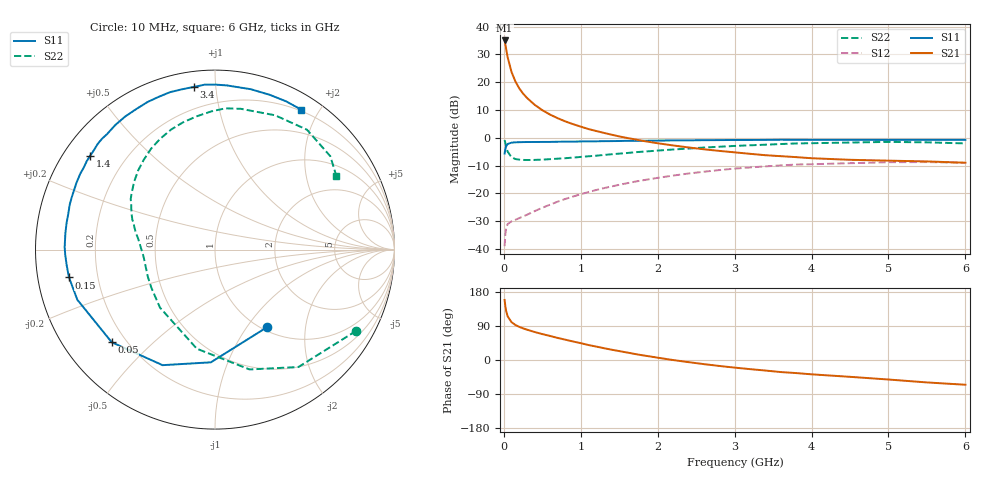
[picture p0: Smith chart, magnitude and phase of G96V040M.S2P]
! SIEMENS Small Signal Semiconductors
! BFG235
! Si NPN RF Bipolar Junction Transistor in SOT223
! VCE = 6 V  IC = 40 mA
! Common Emitter S-Parameters:  July  1994
# GHz  S  MA  R  50
!  f  S11  S21  S12  S22
! GHz  MAG  ANG  MAG  ANG  MAG  ANG  MAG  ANG
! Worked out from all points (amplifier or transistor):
!   40 points, 10 MHz to 6 GHz, reference 50 ohm
!   highest |S21| = 35.0 dB at 10 MHz (marker M1)
!   |S21| within 3 dB of that: start of sweep to 29.72 MHz
!   unconditionally stable (mu >= 1): 522.6 MHz to 1.265 GHz
!   at 200 MHz: K = 0.62, MSG = 23.3 dB, |S12| = -28.9 dB
!   at 1.5 GHz: K = 0.97, MSG = 8.7 dB, |S12| = -16.9 dB
!   at 6 GHz: K = 0.93, MSG = 0.0 dB, |S12| = -9.0 dB
!   S11 on the Smith chart (normalised r, x): 10 MHz: 1.06, -1.25; 50 MHz: 0.15, -0.38; 150 MHz: 0.09, -0.09; 1.4 GHz: 0.08, +0.33; 3.4 GHz: 0.08, +0.88; 6 GHz: 0.18, +1.78
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0.01  0.5206 -56.1  56.27 158.4  0.0112 70.3  0.9077 -29.9
0.02  0.6284 -92.1  47.61 141.4  0.0188 54.8  0.8025 -54.6
0.03  0.707 -114.4  39.63 129.4  0.0235 45.6  0.695 -73.9
0.05  0.773 -138.1  27.87 114.9  0.028 34.4  0.5614 -100.4
0.1  0.8163 -160.0  15.23 99.8  0.0314 28.1  0.4454 -133.5
0.15  0.8282 -169.2  10.31 92.4  0.0334 30.6  0.4137 -148.8
0.2  0.831 -174.0  7.738 87.5  0.0358 33.2  0.404 -157.5
0.25  0.835 -178.0  6.238 83.5  0.0384 36.8  0.3989 -163.1
0.3  0.8377 179.0  5.214 80.1  0.0411 39.3  0.3976 -167.5
0.4  0.8386 173.7  3.925 73.9  0.0478 44.4  0.3991 -173.2
0.5  0.8402 169.8  3.131 68.4  0.055 47.6  0.4042 -177.5
0.6  0.8413 166.4  2.613 63.5  0.0625 49.7  0.4119 179.0
0.7  0.8475 162.7  2.246 58.2  0.0708 51.0  0.4201 175.8
0.9  0.8524 157.0  1.754 48.8  0.0875 51.4  0.4391 170.4
1.1  0.8616 150.6  1.433 39.5  0.1054 50.4  0.4638 165.0
1.4  0.8697 143.1  1.135 27.2  0.1329 46.9  0.5043 157.1
2.2  0.8947 123.9  0.727 -0.1  0.2086 31.8  0.6144 134.2
3.2  0.9118 101.6  0.514 -24.1  0.2921 7.8  0.7307 104.2
3.4  0.9142 97.3  0.485 -27.8  0.3054 2.6  0.7497 97.8
4.5  0.9155 77.4  0.401 -44.4  0.3483 -23.9  0.8198 65.9
5.5  0.9161 64.4  0.375 -59.2  0.3648 -46.7  0.8267 39.0
6  0.916 58.3  0.355 -65.3  0.3533 -55.0  0.7908 31.3
